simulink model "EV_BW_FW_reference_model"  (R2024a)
settings: Solver=VariableStepAuto  StartTime=0.0  StopTime=t_sim  RelTol=1e-3
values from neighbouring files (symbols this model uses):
  A_f = 2.15    [prediction_model_test.m]    (also in main_BW_FW.m; main.m; prediction_longitudinal_model.m; MPC_and_plant_params.m)
  alpha = 0*pi/180    (= 0)    [prediction_model_test.m]    (also in main_BW_FW.m; main.m; prediction_longitudinal_model.m; MPC_and_plant_params.m)
  C_d = 0.33    [prediction_model_test.m]    (also in main_BW_FW.m; main.m; prediction_longitudinal_model.m; MPC_and_plant_params.m)
  eff = Efficiency/100    [main_BW_FW.m]    (also in polinomial_fits.m = e; eff_poly.m = e; main.m; MPC_and_plant_params.m)
  f_0 = 4.5/1000    (= 0.0045)    [prediction_model_test.m]    (also in main_BW_FW.m; main.m; prediction_longitudinal_model.m; MPC_and_plant_params.m)
  g = 9.81    [prediction_model_test.m]    (also in main_BW_FW.m; main.m; prediction_longitudinal_model.m; MPC_and_plant_params.m)
  k = 0    [prediction_model_test.m]    (also in main_BW_FW.m; main.m; prediction_longitudinal_model.m; MPC_and_plant_params.m)
  M_veh = 1400    [prediction_model_test.m]    (also in main_BW_FW.m; main.m; prediction_longitudinal_model.m; MPC_and_plant_params.m)
  N_p = 1    [prediction_model_test.m]    (also in main_BW_FW.m; main.m; prediction_longitudinal_model.m; MPC_and_plant_params.m)
  N_s = 108    [prediction_model_test.m]    (also in main_BW_FW.m; main.m; prediction_longitudinal_model.m; MPC_and_plant_params.m)
  r_w = 0.3    [prediction_model_test.m]    (also in main_BW_FW.m; main.m; prediction_longitudinal_model.m; MPC_and_plant_params.m)
  rho = 1.25    [prediction_model_test.m]    (also in main_BW_FW.m; main.m; prediction_longitudinal_model.m; MPC_and_plant_params.m)
  Ro_s = F_Ro_s(SOC_vec)    [main_BW_FW.m]    (also in main.m; MPC_and_plant_params.m)
  s = tf('s')    [main.m]    (also in MPC_and_plant_params.m; polinomial_fits.m = size(Speed))
  SOC0 = 0.8    [prediction_model_test.m]    (also in main_BW_FW.m; main.m; MPC_and_plant_params.m)
  SOC_vec = linspace(0,1,500)    [main_BW_FW.m]    (also in main.m; MPC_and_plant_params.m)
  tau_gb = 9.6    [prediction_model_test.m]    (also in main_BW_FW.m; main.m; prediction_longitudinal_model.m; MPC_and_plant_params.m)
  Voc_s = F_Voc_s(SOC_vec)    [main_BW_FW.m]    (also in main.m; MPC_and_plant_params.m)
undefined symbols (not defined in the file or in its folder): flip, m, seconds, Shaft_Torque, Speed
libraries: autolibshared x1

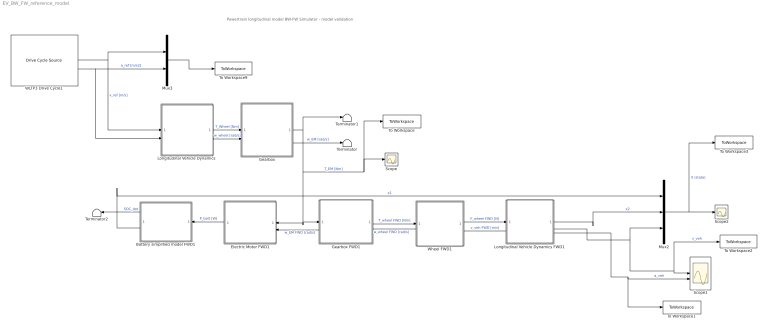
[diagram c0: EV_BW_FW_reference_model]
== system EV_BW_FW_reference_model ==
  note: Powertrain longitudinal model BW-FW Simulator - model validation
  Battery simplified model FWD1 : Subsystem
  Electric Motor FWD1 : Subsystem
  Gearbox : Subsystem
  Gearbox FWD1 : Subsystem
  Longitudinal Vehicle Dynamics : Subsystem
  Longitudinal Vehicle Dynamics FWD1 : Subsystem
  Mux2 : Mux  Inputs=3
  Mux3 : Mux  Inputs=2
  Scope : Scope
  Scope1 : Scope  NumInputPorts=2
  Scope2 : Scope
  Terminator : Terminator
  Terminator1 : Terminator
  Terminator2 : Terminator
  To Workspace : ToWorkspace  VariableName=T_EM_ref  SaveFormat=Timeseries  SampleTime=-1
  To Workspace1 : ToWorkspace  VariableName=a_ref  SaveFormat=Timeseries  SampleTime=-1
  To Workspace2 : ToWorkspace  VariableName=v_val_model  SaveFormat=Timeseries  SampleTime=-1
  To Workspace3 : ToWorkspace  VariableName=X_ref  SaveFormat=Timeseries  SampleTime=-1
  To Workspace9 : ToWorkspace  VariableName=ref  SaveFormat=Timeseries  SampleTime=-1
  WLTP3 Drive Cycle1 : autolibshared/Drive Cycle Source  cycleVar=Workspace variable  wsVar=vehspeed  fileVar=cycleFTP75.mat  tfinal="1800  seconds"  cycleRepeat=off  outAccPort=on  outGearPort=off  gearList=No gear data  t_wot1=5  xdot_woto=0  xdot_wot1=30  t_wot2=20  xdot_wot2=0  t_wotend=30  srcUnit=m/s  outUnit=m/s  srcAccUnit=m/s/s  outAccUnit=m/s^2  dt=0  aMode=1  faultOption=off  velBnd=2  velBndUnit=mph  inUnit=m/s  timeBnd=1  failOption=off  stopSim=off  maxFaultCnt=10  maxFaultTime=2  maxTotFaultTime=15  traceOption=off  dtTrace=1  traceWindow=10  lastDCname=Custom Data Set  lastOutUnit=mph  lastDT=0  lastTB=1  lastSB=2  forceCalcBound=off
  Wheel FWD1 : Subsystem
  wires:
  Battery simplified model FWD1/2(SOC) -> Mux2/1  "x1"
  Battery simplified model FWD1/1(SOC_dot) -> Terminator2/1  "SOC_dot"
  Mux3/1 -> To Workspace9/1
  Mux2/1 -> To Workspace3/1, Scope2/1  "X (state)"
  Longitudinal Vehicle Dynamics FWD1/4(v_veh1) -> Wheel FWD1/2(v_veh)  "v_veh FWD [m/s]"
  Electric Motor FWD1/1(P_batt) -> Battery simplified model FWD1/1(P_batt)  "P_batt [W]"
  Longitudinal Vehicle Dynamics FWD1/2(v_veh) -> To Workspace2/1, Scope1/1, Mux2/3  "v_veh"
  Longitudinal Vehicle Dynamics FWD1/1("x_veh ") -> Mux2/2  "x2"
  Gearbox FWD1/1(T_wheel) -> Wheel FWD1/1(T_wheel)  "T_wheel FWD [Nm]"
  Wheel FWD1/2(w_wheel) -> Gearbox FWD1/2(w_wheel)  "w_wheel FWD [rad/s]"
  Gearbox FWD1/2(w_EM) -> Electric Motor FWD1/2(w_EM)  "w_EM FWD [rad/s]"
  Wheel FWD1/1(F_wheel) -> Longitudinal Vehicle Dynamics FWD1/1(F_trac)  "F_wheel FWD [N]"
  Longitudinal Vehicle Dynamics/2(w_wheel) -> Gearbox/2(w_wheel)  "w_wheel [rad/s]"
  Longitudinal Vehicle Dynamics/1(T_wheel) -> Gearbox/1(T_wheel)  "T_Wheel [Nm]"
  WLTP3 Drive Cycle1/2 -> Longitudinal Vehicle Dynamics/2(a_ref), Mux3/2  "a_ref [m/s2]"
  Gearbox/2(w_EM) -> Terminator/1  "w_EM [rad/s]"
  WLTP3 Drive Cycle1/1 -> Longitudinal Vehicle Dynamics/1(v_ref), Mux3/1  "v_ref [m/s]"
  Gearbox/1(T_EM) -> Electric Motor FWD1/1(T_EM), Gearbox FWD1/1(T_EM), To Workspace/1, Scope/1, Terminator1/1  "T_EM [Nm]"
  Longitudinal Vehicle Dynamics FWD1/3(a_veh) -> To Workspace1/1, Scope1/2  "a_veh"

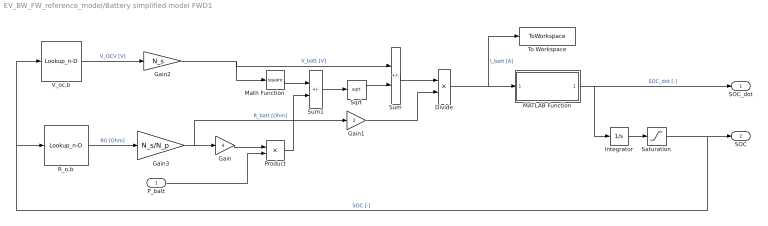
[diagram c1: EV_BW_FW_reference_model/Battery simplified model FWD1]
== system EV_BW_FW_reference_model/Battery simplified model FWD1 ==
  P_batt : Inport
  Divide : Product  Inputs=*/
  Gain : Gain  Gain=4
  Gain1 : Gain  Gain=2
  Gain2 : Gain  Gain=N_s
  Gain3 : Gain  Gain=N_s/N_p
  Integrator : Integrator  InitialCondition=SOC0
  MATLAB Function : MATLAB Function  TreatAsAtomicUnit=on
  Math Function : Math  Operator=square
  Product : Product
  R_o,b : Lookup_n-D  NumberOfTableDimensions=1  BreakpointsForDimension1=SOC_vec  BreakpointsForDimension3=[5, 7]  Table=Ro_s  InternalRulePriority=Speed  RndMeth=Simplest
  Saturation : Saturate  UpperLimit=1  LowerLimit=0
  Sqrt : Sqrt
  Sum : Sum  Inputs=+-
  Sum1 : Sum  Inputs=+-
  To Workspace : ToWorkspace  VariableName=Ib_controlled  SaveFormat=Timeseries  SampleTime=-1
  V_oc,b : Lookup_n-D  NumberOfTableDimensions=1  BreakpointsForDimension1=SOC_vec  BreakpointsForDimension3=[5, 7]  Table=Voc_s  InternalRulePriority=Speed  RndMeth=Simplest
  SOC_dot : Outport
  SOC : Outport  Port=2
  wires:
  Math Function/1 -> Sum1/1
  Gain/1 -> Product/1
  Product/1 -> Sum1/2
  Sum1/1 -> Sqrt/1
  Sqrt/1 -> Sum/2
  Sum/1 -> Divide/1
  Gain1/1 -> Divide/2
  Divide/1 -> MATLAB Function/1(I_b), To Workspace/1  "I_batt [A]"
  MATLAB Function/1(SOC_dot) -> SOC_dot/1, Integrator/1  "SOC_dot [-]"
  Integrator/1 -> Saturation/1
  R_o,b/1 -> Gain3/1  "R0 [Ohm]"
  V_oc,b/1 -> Gain2/1  "V_OCV [V]"
  Gain2/1 -> Sum/1, Math Function/1  "V_batt [V]"
  Gain3/1 -> Gain1/1, Gain/1  "R_batt [Ohm]"
  Saturation/1 -> V_oc,b/1, R_o,b/1, SOC/1  "SOC [-]"
  P_batt/1 -> Product/2

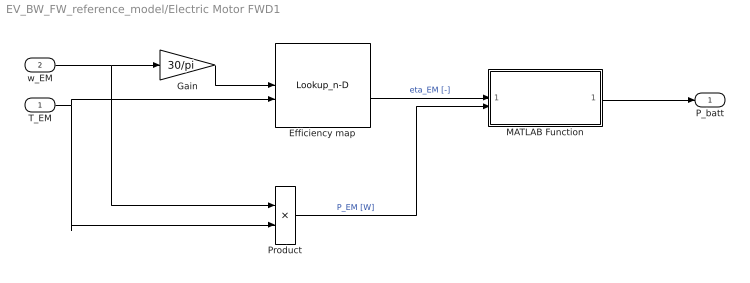
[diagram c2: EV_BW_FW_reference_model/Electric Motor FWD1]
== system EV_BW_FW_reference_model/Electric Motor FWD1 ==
  T_EM : Inport
  w_EM : Inport  Port=2
  Efficiency map : Lookup_n-D  BreakpointsForDimension1=Speed(:,1)  BreakpointsForDimension2=flip(Shaft_Torque(1,:))  BreakpointsForDimension3=[5, 7]  Table=flip(eff)  InternalRulePriority=Speed  RndMeth=Simplest
  Gain : Gain  Gain=30/pi
  MATLAB Function : MATLAB Function  TreatAsAtomicUnit=on
  Product : Product
  P_batt : Outport
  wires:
  w_EM/1 -> Gain/1, Product/1
  T_EM/1 -> Efficiency map/2, Product/2
  Product/1 -> MATLAB Function/2(P_EM)  "P_EM [W]"
  MATLAB Function/1(P_batt) -> P_batt/1
  Efficiency map/1 -> MATLAB Function/1(eta_EM)  "eta_EM [-]"
  Gain/1 -> Efficiency map/1

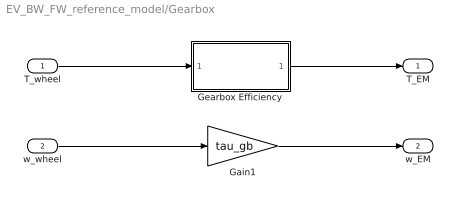
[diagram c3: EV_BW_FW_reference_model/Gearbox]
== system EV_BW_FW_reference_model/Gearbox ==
  T_wheel : Inport
  w_wheel : Inport  Port=2
  Gain1 : Gain  Gain=tau_gb
  Gearbox Efficiency : MATLAB Function  TreatAsAtomicUnit=on
  T_EM : Outport
  w_EM : Outport  Port=2
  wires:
  Gain1/1 -> w_EM/1
  Gearbox Efficiency/1(T_EM) -> T_EM/1
  T_wheel/1 -> Gearbox Efficiency/1(T_out)
  w_wheel/1 -> Gain1/1

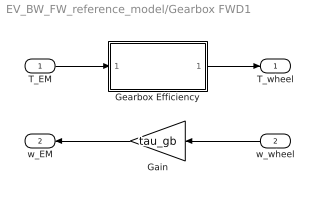
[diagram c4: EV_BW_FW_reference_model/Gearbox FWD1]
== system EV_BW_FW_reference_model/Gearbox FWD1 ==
  T_EM : Inport
  w_wheel : Inport  Port=2
  Gain : Gain  Gain=tau_gb
  Gearbox Efficiency : MATLAB Function  TreatAsAtomicUnit=on
  T_wheel : Outport
  w_EM : Outport  Port=2
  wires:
  T_EM/1 -> Gearbox Efficiency/1(T_EM)
  Gearbox Efficiency/1(T_wheel) -> T_wheel/1
  w_wheel/1 -> Gain/1
  Gain/1 -> w_EM/1

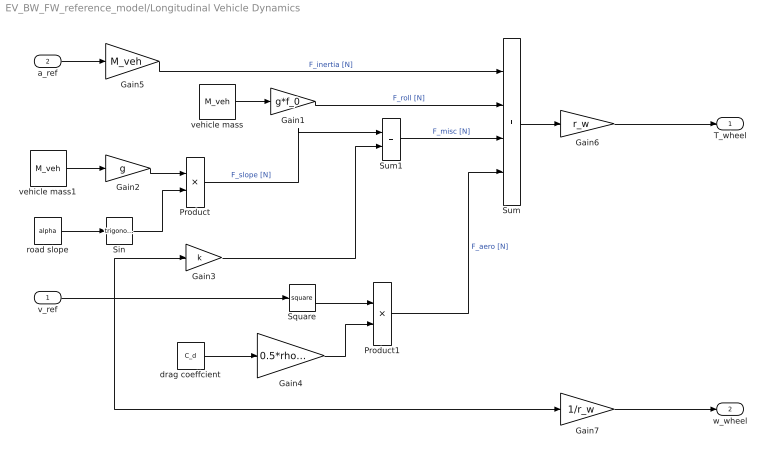
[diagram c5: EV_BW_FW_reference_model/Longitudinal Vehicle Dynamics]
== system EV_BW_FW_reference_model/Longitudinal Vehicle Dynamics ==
  v_ref : Inport
  a_ref : Inport  Port=2
  Gain1 : Gain  Gain=g*f_0
  Gain2 : Gain  Gain=g
  Gain3 : Gain  Gain=k
  Gain4 : Gain  Gain=0.5*rho*A_f
  Gain5 : Gain  Gain=M_veh
  Gain6 : Gain  Gain=r_w
  Gain7 : Gain  Gain=1/r_w
  Product : Product
  Product1 : Product
  Sin : Trigonometry
  Square : Math  Operator=square
  Sum : Sum  Inputs=++++
  Sum1 : Sum
  drag coeffcient : Constant  Value=C_d
  road slope : Constant  Value=alpha
  vehicle mass : Constant  Value=M_veh
  vehicle mass1 : Constant  Value=M_veh
  T_wheel : Outport
  w_wheel : Outport  Port=2
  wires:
  drag coeffcient/1 -> Gain4/1
  Gain4/1 -> Product1/2
  Sum1/1 -> Sum/3  "F_misc [N]"
  Gain2/1 -> Product/1
  vehicle mass/1 -> Gain1/1
  Gain1/1 -> Sum/2  "F_roll [N]"
  Square/1 -> Product1/1
  vehicle mass1/1 -> Gain2/1
  road slope/1 -> Sin/1
  Gain5/1 -> Sum/1  "F_inertia [N]"
  Product1/1 -> Sum/4  "F_aero [N]"
  Sin/1 -> Product/2
  Gain6/1 -> T_wheel/1
  Product/1 -> Sum1/1  "F_slope [N]"
  Gain3/1 -> Sum1/2
  Sum/1 -> Gain6/1
  a_ref/1 -> Gain5/1
  v_ref/1 -> Gain7/1, Gain3/1, Square/1
  Gain7/1 -> w_wheel/1

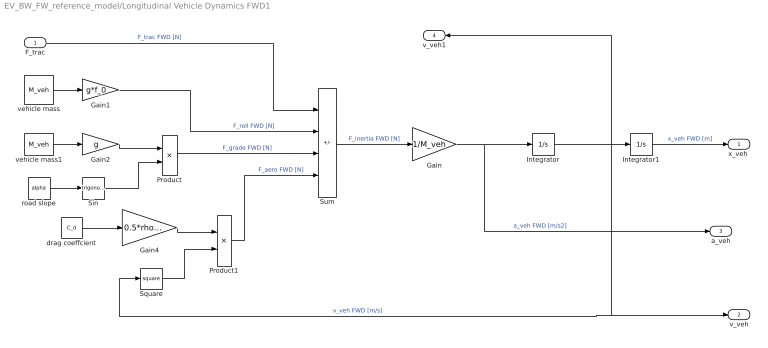
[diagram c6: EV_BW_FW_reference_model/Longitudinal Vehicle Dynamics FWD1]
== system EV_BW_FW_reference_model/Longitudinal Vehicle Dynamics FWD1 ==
  F_trac : Inport
  Gain : Gain  Gain=1/M_veh
  Gain1 : Gain  Gain=g*f_0
  Gain2 : Gain  Gain=g
  Gain4 : Gain  Gain=0.5*rho*A_f
  Integrator : Integrator
  Integrator1 : Integrator
  Product : Product
  Product1 : Product
  Sin : Trigonometry
  Square : Math  Operator=square
  Sum : Sum  Inputs=+---
  drag coeffcient : Constant  Value=C_d
  road slope : Constant  Value=alpha
  vehicle mass : Constant  Value=M_veh
  vehicle mass1 : Constant  Value=M_veh
  "x_veh " : Outport
  v_veh : Outport  Port=2
  a_veh : Outport  Port=3
  v_veh1 : Outport  Port=4
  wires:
  drag coeffcient/1 -> Gain4/1
  Gain2/1 -> Product/1
  vehicle mass/1 -> Gain1/1
  Gain1/1 -> Sum/2  "F_roll FWD [N]"
  vehicle mass1/1 -> Gain2/1
  road slope/1 -> Sin/1
  Product1/1 -> Sum/4  "F_aero FWD [N]"
  Sin/1 -> Product/2
  Product/1 -> Sum/3  "F_grade FWD [N]"
  F_trac/1 -> Sum/1  "F_trac FWD [N]"
  Gain4/1 -> Product1/1
  Square/1 -> Product1/2
  Sum/1 -> Gain/1  "F_inertia FWD [N]"
  Gain/1 -> a_veh/1, Integrator/1  "a_veh FWD [m/s2]"
  Integrator/1 -> Square/1, v_veh/1, v_veh1/1, Integrator1/1  "v_veh FWD [m/s]"
  Integrator1/1 -> "x_veh "/1  "x_veh FWD [m]"

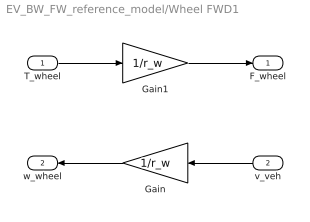
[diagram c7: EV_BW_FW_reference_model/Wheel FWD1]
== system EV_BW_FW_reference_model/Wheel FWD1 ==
  T_wheel : Inport
  v_veh : Inport  Port=2
  Gain : Gain  Gain=1/r_w
  Gain1 : Gain  Gain=1/r_w
  F_wheel : Outport
  w_wheel : Outport  Port=2
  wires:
  T_wheel/1 -> Gain1/1
  Gain1/1 -> F_wheel/1
  v_veh/1 -> Gain/1
  Gain/1 -> w_wheel/1

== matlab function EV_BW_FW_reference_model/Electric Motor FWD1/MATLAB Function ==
function P_batt = fcn(eta_EM,P_EM)
eta_inv = 1;

P_batt = P_EM/((eta_EM*eta_inv)^(sign(P_EM)));

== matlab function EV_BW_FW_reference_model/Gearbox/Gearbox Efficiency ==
function T_EM = fcn(T_out)
eta_gb = 0.97;
tau_gb = 9.6;

T_EM = T_out/(tau_gb*eta_gb^(sign(T_out)));

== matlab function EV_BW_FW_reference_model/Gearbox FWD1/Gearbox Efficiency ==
function T_wheel = fcn(T_EM)
eta_gb = 0.97;
tau_gb = 9.6;

T_wheel = T_EM * ((tau_gb*eta_gb^(sign(T_EM))));

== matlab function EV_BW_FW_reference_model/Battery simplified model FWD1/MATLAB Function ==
function SOC_dot = fcn(I_b)
    eta_c = 0.95;
    Q_nom = 60*1*3600;
    if I_b > 0 % discharge
        SOC_dot = -I_b/(eta_c*Q_nom);
    else % charge
        SOC_dot = -eta_c*I_b/Q_nom;
    end
